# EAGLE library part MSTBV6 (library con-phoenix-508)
PHOENIX
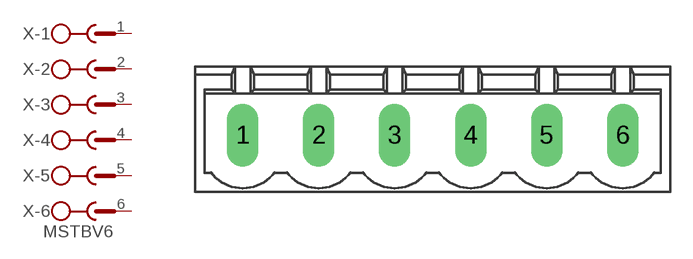
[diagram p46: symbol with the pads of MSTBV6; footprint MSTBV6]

Designator prefix X; gates -1=SK -2=SK -3=SK -4=SK -5=SK -6=SKV

## MSTBV6 (MPN: MSTBV 2,5/6-GF-5.08; OC_FARNELL: 1792796; OC_NEWARK: 69R9849)  [MSTBV6]
1  -1:1  pas
2  -2:1  pas
3  -3:1  pas
4  -4:1  pas
5  -5:1  pas
6  -6:1  pas

## Footprint MSTBV6 (pad centres in mm)
PHOENIX
drill 1.397 long: 1 -12.7,0; 2 -7.62,0; 3 -2.54,0; 4 2.54,0; 5 7.62,0; 6 12.7,0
